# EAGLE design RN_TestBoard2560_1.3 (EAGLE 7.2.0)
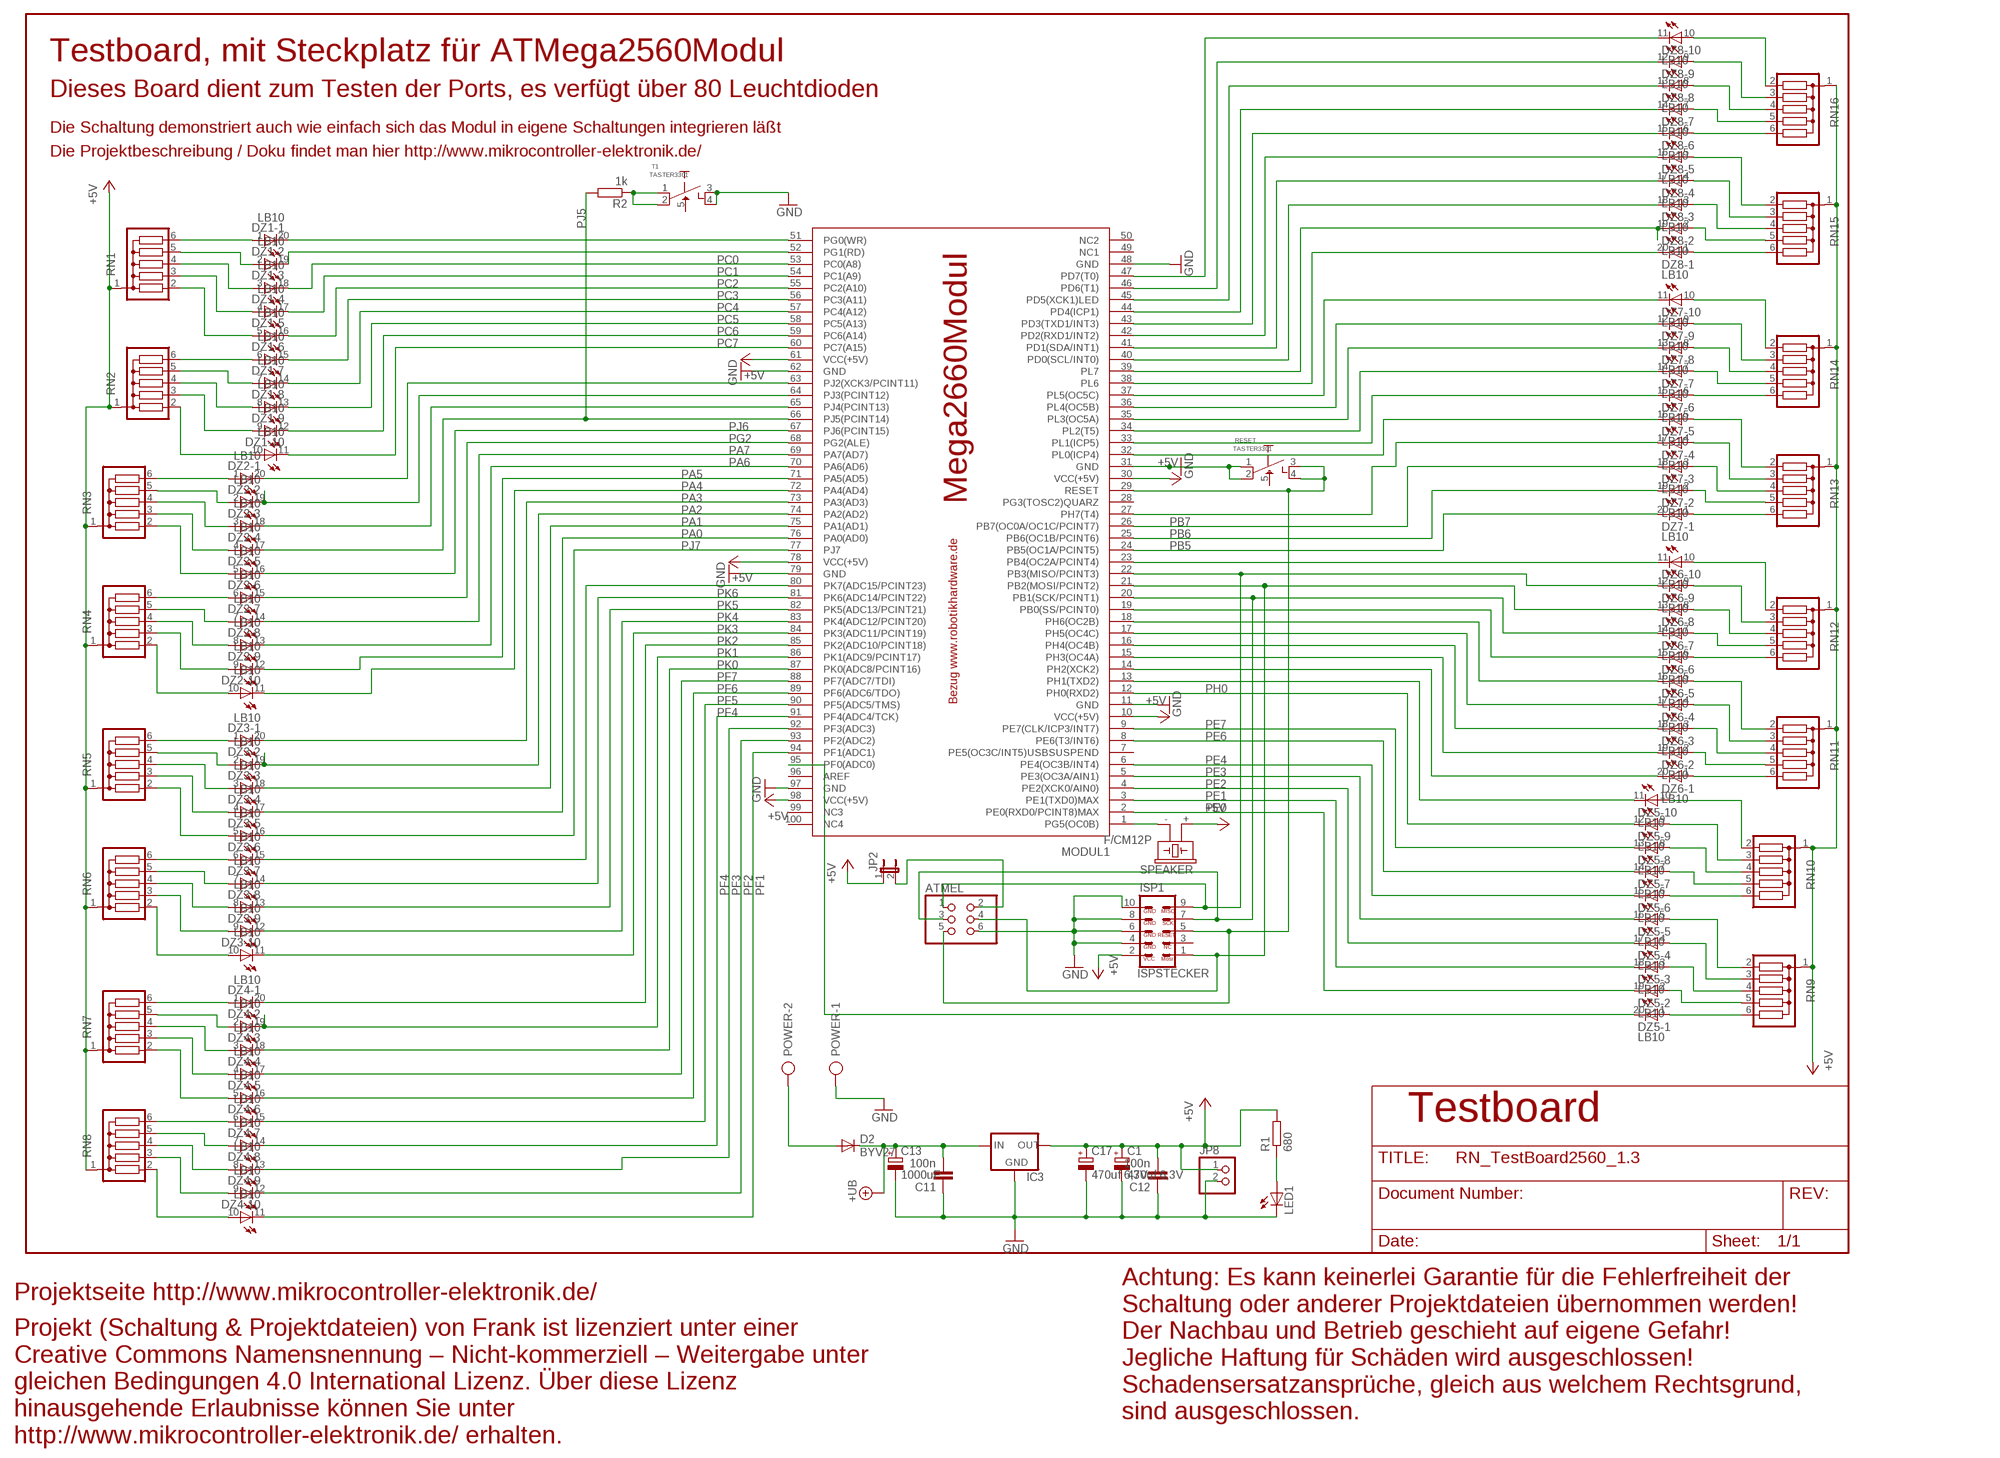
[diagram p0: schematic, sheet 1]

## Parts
ATMEL  PINHD-2X3  [2X03]
C1  470uf 6,3V  CPOL-EUE3.5-8  [E3,5-8]
C11  100n  C-EU050-024X044  [C050-024X044]
C12  100n  C-EU050-024X044  [C050-024X044]
C13  1000uF  CPOL-EUE5-13  [E5-13]
C17  470uf 6,3V  CPOL-EUE3.5-8  [E3,5-8]
D2  BYV27  [SOD57-10]
DZ1  LB10  [LB10]
DZ2  LB10  [LB10]
DZ3  LB10  [LB10]
DZ4  LB10  [LB10]
DZ5  LB10  [LB10]
DZ6  LB10  [LB10]
DZ7  LB10  [LB10]
DZ8  LB10  [LB10]
IC3  78XXS  [78XXS]
ISP1  ISPSTECKER  [ML10]
JP2  JP1E  [JP1]
JP8  PINHD-1X2  [1X02]
LED1  LED3MM  [LED3MM]
MODUL1  MEGA2560MODUL  [MEGA2560MODUL]
POWER  AK500/2  [AK500/2]
R1  680  R-EU_0207/10  [0207/10]
R2  1k  R-EU_0207/10  [0207/10]
RESET  TASTER3301  [TASTER]
RN1  G05R  [SIL6]
RN2  G05R  [SIL6]
RN3  G05R  [SIL6]
RN4  G05R  [SIL6]
RN5  G05R  [SIL6]
RN6  G05R  [SIL6]
RN7  G05R  [SIL6]
RN8  G05R  [SIL6]
RN9  G05R  [SIL6]
RN10  G05R  [SIL6]
RN11  G05R  [SIL6]
RN12  G05R  [SIL6]
RN13  G05R  [SIL6]
RN14  G05R  [SIL6]
RN15  G05R  [SIL6]
RN16  G05R  [SIL6]
SPEAKER  F/CM12P  [F/CM12P]
T1  TASTER3301  [TASTER]

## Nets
+5V [Power3A]: C1.+ C12.2 C17.+ IC3.OUT ISP1.2 JP2.1 JP8.1 MODUL1.10(VCC(+5V)) MODUL1.30(VCC(+5V)) MODUL1.61(VCC(+5V)) MODUL1.78(VCC(+5V)) MODUL1.98(VCC(+5V)) R1.2 RN1.1 RN2.1 RN3.1 RN4.1 RN5.1 RN6.1 RN7.1 RN8.1 RN9.1 RN10.1 RN11.1 RN12.1 RN13.1 RN14.1 RN15.1 RN16.1 SPEAKER.+
+UB [Power2A]: C11.2 C13.+ D2.C IC3.IN
GND [Power2A]: ATMEL.6 C1.- C11.1 C12.1 C13.- C17.- IC3.GND ISP1.4 ISP1.6 ISP1.8 ISP1.10 JP8.2 LED1.K(C) MODUL1.11(GND) MODUL1.31(GND) MODUL1.48(GND) MODUL1.62(GND) MODUL1.79(GND) MODUL1.97(GND) POWER.1 RESET.1 RESET.2 T1.3 T1.4
N$1: ATMEL.2 JP2.2
N$2: ATMEL.5 ISP1.5 MODUL1.29(RESET) RESET.3 RESET.4
N$3: DZ5.20(-1:C) MODUL1.95(PF0(ADC0))
N$4: LED1.A R1.1
N$5: R2.1 T1.1 T1.2
N$9: DZ1.1(-1:A) RN1.6
N$10: DZ1.2(-2:A) RN1.5
N$11: DZ1.3(-3:A) RN1.4
N$12: DZ1.4(-4:A) RN1.3
N$13: DZ1.5(-5:A) RN1.2
N$14: DZ1.6(-6:A) RN2.6
N$15: DZ1.7(-7:A) RN2.5
N$16: DZ1.8(-8:A) RN2.4
N$17: DZ1.9(-9:A) RN2.3
N$18: DZ1.10(-10:A) RN2.2
N$19: DZ1.20(-1:C) MODUL1.51(PG0(WR))
N$20: DZ1.19(-2:C) MODUL1.52(PG1(RD))
N$29: DZ2.3(-3:A) RN3.4
N$30: DZ2.4(-4:A) RN3.3
N$31: DZ2.5(-5:A) RN3.2
N$32: DZ2.7(-7:A) RN4.5
N$33: DZ2.8(-8:A) RN4.4
N$34: DZ2.9(-9:A) RN4.3
N$35: DZ2.10(-10:A) RN4.2
N$36: DZ2.18(-3:C) MODUL1.65(PJ4(PCINT13))
N$37: D2.A POWER.2
N$45: DZ2.1(-1:A) RN3.6
N$46: DZ2.2(-2:A) RN3.5
N$47: DZ2.6(-6:A) RN4.6
N$48: DZ2.20(-1:C) MODUL1.63(PJ2(XCK3/PCINT11))
N$49: DZ2.19(-2:C) MODUL1.64(PJ3(PCINT12))
N$50: DZ8.16(-5:C) MODUL1.42(PD2(RXD1/INT2))
N$52: DZ5.3(-3:A) RN9.4
N$53: DZ5.4(-4:A) RN9.3
N$54: DZ5.5(-5:A) RN9.2
N$55: DZ5.7(-7:A) RN10.5
N$56: DZ5.8(-8:A) RN10.4
N$57: MODUL1.1(PG5(OC0B)) SPEAKER.-
N$58: DZ5.9(-9:A) RN10.3
N$59: DZ3.3(-3:A) RN5.4
N$60: DZ3.4(-4:A) RN5.3
N$61: DZ3.5(-5:A) RN5.2
N$62: DZ3.7(-7:A) RN6.5
N$63: DZ3.8(-8:A) RN6.4
N$64: DZ3.9(-9:A) RN6.3
N$65: DZ3.10(-10:A) RN6.2
N$69: DZ3.15(-6:C) MODUL1.80(PK7(ADC15/PCINT23))
N$74: DZ3.1(-1:A) RN5.6
N$75: DZ3.2(-2:A) RN5.5
N$76: DZ3.6(-6:A) RN6.6
N$79: DZ5.10(-10:A) RN10.2
N$86: DZ5.11(-10:C) MODUL1.13(PH1(TXD2))
N$87: DZ6.20(-1:C) MODUL1.14(PH2(XCK2))
N$88: DZ5.1(-1:A) RN9.6
N$89: DZ4.3(-3:A) RN7.4
N$90: DZ4.4(-4:A) RN7.3
N$91: DZ4.5(-5:A) RN7.2
N$92: DZ4.7(-7:A) RN8.5
N$93: DZ4.8(-8:A) RN8.4
N$94: DZ4.9(-9:A) RN8.3
N$95: DZ4.10(-10:A) RN8.2
N$104: DZ4.1(-1:A) RN7.6
N$105: DZ4.2(-2:A) RN7.5
N$106: DZ4.6(-6:A) RN8.6
N$109: DZ5.2(-2:A) RN9.5
N$110: DZ5.6(-6:A) RN10.6
N$113: DZ6.3(-3:A) RN11.4
N$114: DZ6.4(-4:A) RN11.3
N$115: DZ6.5(-5:A) RN11.2
N$116: DZ6.7(-7:A) RN12.5
N$117: DZ6.8(-8:A) RN12.4
N$118: DZ6.9(-9:A) RN12.3
N$119: DZ6.10(-10:A) RN12.2
N$120: DZ6.17(-4:C) MODUL1.17(PH5(OC4C))
N$121: DZ6.16(-5:C) MODUL1.18(PH6(OC2B))
N$122: DZ6.15(-6:C) MODUL1.19(PB0(SS/PCINT0))
N$123: ATMEL.3 DZ6.14(-7:C) ISP1.7 MODUL1.20(PB1(SCK/PCINT1))
N$124: ATMEL.4 DZ6.13(-8:C) ISP1.1 MODUL1.21(PB2(MOSI/PCINT2))
N$125: ATMEL.1 DZ6.12(-9:C) ISP1.9 MODUL1.22(PB3(MISO/PCINT3))
N$126: DZ6.11(-10:C) MODUL1.23(PB4(OC2A/PCINT4))
N$128: DZ6.1(-1:A) RN11.6
N$129: DZ6.2(-2:A) RN11.5
N$130: DZ6.6(-6:A) RN12.6
N$131: DZ6.18(-3:C) MODUL1.16(PH4(OC4B))
N$132: DZ6.19(-2:C) MODUL1.15(PH3(OC4A))
N$133: DZ7.3(-3:A) RN13.4
N$134: DZ7.4(-4:A) RN13.3
N$135: DZ7.5(-5:A) RN13.2
N$136: DZ7.7(-7:A) RN14.5
N$137: DZ7.8(-8:A) RN14.4
N$138: DZ7.9(-9:A) RN14.3
N$139: DZ7.10(-10:A) RN14.2
N$140: DZ7.17(-4:C) MODUL1.27(PH7(T4))
N$142: DZ7.16(-5:C) MODUL1.32(PL0(ICP4))
N$143: DZ7.15(-6:C) MODUL1.33(PL1(ICP5))
N$144: DZ7.14(-7:C) MODUL1.34(PL2(T5))
N$145: DZ7.13(-8:C) MODUL1.35(PL3(OC5A))
N$146: DZ7.12(-9:C) MODUL1.36(PL4(OC5B))
N$147: DZ7.11(-10:C) MODUL1.37(PL5(OC5C))
N$148: DZ7.1(-1:A) RN13.6
N$149: DZ7.2(-2:A) RN13.5
N$150: DZ7.6(-6:A) RN14.6
N$153: DZ8.3(-3:A) RN15.4
N$154: DZ8.4(-4:A) RN15.3
N$155: DZ8.5(-5:A) RN15.2
N$156: DZ8.7(-7:A) RN16.5
N$157: DZ8.8(-8:A) RN16.4
N$158: DZ8.9(-9:A) RN16.3
N$159: DZ8.10(-10:A) RN16.2
N$160: DZ8.18(-3:C) MODUL1.40(PD0(SCL/INT0))
N$161: DZ8.17(-4:C) MODUL1.41(PD1(SDA/INT1))
N$163: DZ8.15(-6:C) MODUL1.43(PD3(TXD1/INT3))
N$164: DZ8.14(-7:C) MODUL1.44(PD4(ICP1))
N$165: DZ8.13(-8:C) MODUL1.45(PD5(XCK1)LED)
N$166: DZ8.12(-9:C) MODUL1.46(PD6(T1))
N$167: DZ8.11(-10:C) MODUL1.47(PD7(T0))
N$168: DZ8.1(-1:A) RN15.6
N$169: DZ8.2(-2:A) RN15.5
N$170: DZ8.6(-6:A) RN16.6
N$171: DZ8.19(-2:C) MODUL1.39(PL7)
N$172: DZ8.20(-1:C) MODUL1.38(PL6)
PA0: DZ3.17(-4:C) MODUL1.76(PA0(AD0))
PA1: DZ3.18(-3:C) MODUL1.75(PA1(AD1))
PA2: DZ3.19(-2:C) MODUL1.74(PA2(AD2))
PA3: DZ3.20(-1:C) MODUL1.73(PA3(AD3))
PA4: DZ2.11(-10:C) MODUL1.72(PA4(AD4))
PA5: DZ2.12(-9:C) MODUL1.71(PA5(AD5))
PA6: DZ2.13(-8:C) MODUL1.70(PA6(AD6))
PA7: DZ2.14(-7:C) MODUL1.69(PA7(AD7))
PB5: DZ7.20(-1:C) MODUL1.24(PB5(OC1A/PCINT5))
PB6: DZ7.19(-2:C) MODUL1.25(PB6(OC1B/PCINT6))
PB7: DZ7.18(-3:C) MODUL1.26(PB7(OC0A/OC1C/PCINT7))
PC0: DZ1.18(-3:C) MODUL1.53(PC0(A8))
PC1: DZ1.17(-4:C) MODUL1.54(PC1(A9))
PC2: DZ1.16(-5:C) MODUL1.55(PC2(A10))
PC3: DZ1.15(-6:C) MODUL1.56(PC3(A11))
PC4: DZ1.14(-7:C) MODUL1.57(PC4(A12))
PC5: DZ1.13(-8:C) MODUL1.58(PC5(A13))
PC6: DZ1.12(-9:C) MODUL1.59(PC6(A14))
PC7: DZ1.11(-10:C) MODUL1.60(PC7(A15))
PE0: DZ5.19(-2:C) MODUL1.2(PE0(RXD0/PCINT8)MAX)
PE1: DZ5.18(-3:C) MODUL1.3(PE1(TXD0)MAX)
PE2: DZ5.17(-4:C) MODUL1.4(PE2(XCK0/AIN0))
PE3: DZ5.16(-5:C) MODUL1.5(PE3(OC3A/AIN1))
PE4: DZ5.15(-6:C) MODUL1.6(PE4(OC3B/INT4))
PE6: DZ5.14(-7:C) MODUL1.8(PE6(T3/INT6))
PE7: DZ5.13(-8:C) MODUL1.9(PE7(CLK/ICP3/INT7))
PF1: DZ4.11(-10:C) MODUL1.94(PF1(ADC1))
PF2: DZ4.12(-9:C) MODUL1.93(PF2(ADC2))
PF3: DZ4.13(-8:C) MODUL1.92(PF3(ADC3))
PF4: DZ4.14(-7:C) MODUL1.91(PF4(ADC4/TCK))
PF5: DZ4.15(-6:C) MODUL1.90(PF5(ADC5/TMS))
PF6: DZ4.16(-5:C) MODUL1.89(PF6(ADC6/TDO))
PF7: DZ4.17(-4:C) MODUL1.88(PF7(ADC7/TDI))
PG2: DZ2.15(-6:C) MODUL1.68(PG2(ALE))
PH0: DZ5.12(-9:C) MODUL1.12(PH0(RXD2))
PJ5: DZ2.17(-4:C) MODUL1.66(PJ5(PCINT14)) R2.2
PJ6: DZ2.16(-5:C) MODUL1.67(PJ6(PCINT15))
PJ7: DZ3.16(-5:C) MODUL1.77(PJ7)
PK0: DZ4.18(-3:C) MODUL1.87(PK0(ADC8/PCINT16))
PK1: DZ4.19(-2:C) MODUL1.86(PK1(ADC9/PCINT17))
PK2: DZ4.20(-1:C) MODUL1.85(PK2(ADC10/PCINT18))
PK3: DZ3.11(-10:C) MODUL1.84(PK3(ADC11/PCINT19))
PK4: DZ3.12(-9:C) MODUL1.83(PK4(ADC12/PCINT20))
PK5: DZ3.13(-8:C) MODUL1.82(PK5(ADC13/PCINT21))
PK6: DZ3.14(-7:C) MODUL1.81(PK6(ADC14/PCINT22))
Unconnected: ISP1.3 MODUL1.7(PE5(OC3C/INT5)USBSUSPEND) MODUL1.28(PG3(TOSC2)QUARZ) MODUL1.49(NC1) MODUL1.50(NC2) MODUL1.96(AREF) MODUL1.99(NC3) MODUL1.100(NC4) RESET.5 T1.5

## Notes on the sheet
- Testboard, mit Steckplatz für ATMega2560Modul
- Dieses Board dient zum Testen der Ports, es verfügt über 80 Leuchtdioden
- Die Schaltung demonstriert auch wie einfach sich das Modul in eigene Schaltungen integrieren läßt
- Die Projektbeschreibung / Doku findet man hier http://www.mikrocontroller-elektronik.de/
- Testboard
- Projektseite http://www.mikrocontroller-elektronik.de/
- Achtung: Es kann keinerlei Garantie für die Fehlerfreiheit der
  Schaltung oder anderer Projektdateien übernommen werden!
  Der Nachbau und Betrieb geschieht auf eigene Gefahr! 
  Jegliche Haftung für Schäden wird ausgeschlossen!
  Schadensersatzansprüche, gleich aus welchem Rechtsgrund,
  sind ausgeschlossen.
- Projekt (Schaltung & Projektdateien) von Frank ist lizenziert unter einer
  Creative Commons Namensnennung – Nicht-kommerziell – Weitergabe unter
  gleichen Bedingungen 4.0 International Lizenz. Über diese Lizenz
  hinausgehende Erlaubnisse können Sie unter
  http://www.mikrocontroller-elektronik.de/ erhalten.

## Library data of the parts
ATMEL = pinhead:PINHD-2X3: PIN HEADER
C1 C13 C17 = rcl:CPOL-EU: POLARIZED CAPACITOR, European symbol
C11 C12 = rcl:C-EU: CAPACITOR, European symbol
D2 = diode:BYV27: DIODE
DZ1-DZ8 = led:LB10: LED BLOCK 10-LED bar graph, DIL, Siemens
IC3 = v-reg:78XXS: VOLTAGE REGULATOR
ISP1 = RoboterNetz:ISPSTECKER
JP2 = jumper:JP1E: JUMPER
JP8 = pinhead:PINHD-1X2: PIN HEADER
LED1 = led:LED: LED
MODUL1 = RoboterNetz:MEGA2560MODUL: Sehr kleines Modul mit leistungsstarkem AVR AtMega2560 Controller , RS232 als auch USB - Schnittstelle. Bestückt auch mit Standard ISP Wannenstiftleiste Stecker zum programmieren. Durch modernste SMD Bauteile konnte das Modul so klein gehalten werden. Der Pinabstand der beiden Stiftleisten ist so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
POWER = con-ptr500:AK500/2: CONNECTOR
R1 R2 = rcl:R-EU_: RESISTOR, European symbol
RESET T1 = RoboterNetz:TASTER3301: Taster 3301 Bezugsquelle z.B. Reichelt
RN1-RN16 = resistor-sil:G05R: SIL RESISTOR
SPEAKER = buzzer:F/CM12P: BUZZER

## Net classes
1 power: width 0.457 mm
2 Power2A: width 0.762 mm
3 Power3A: width 1.016 mm

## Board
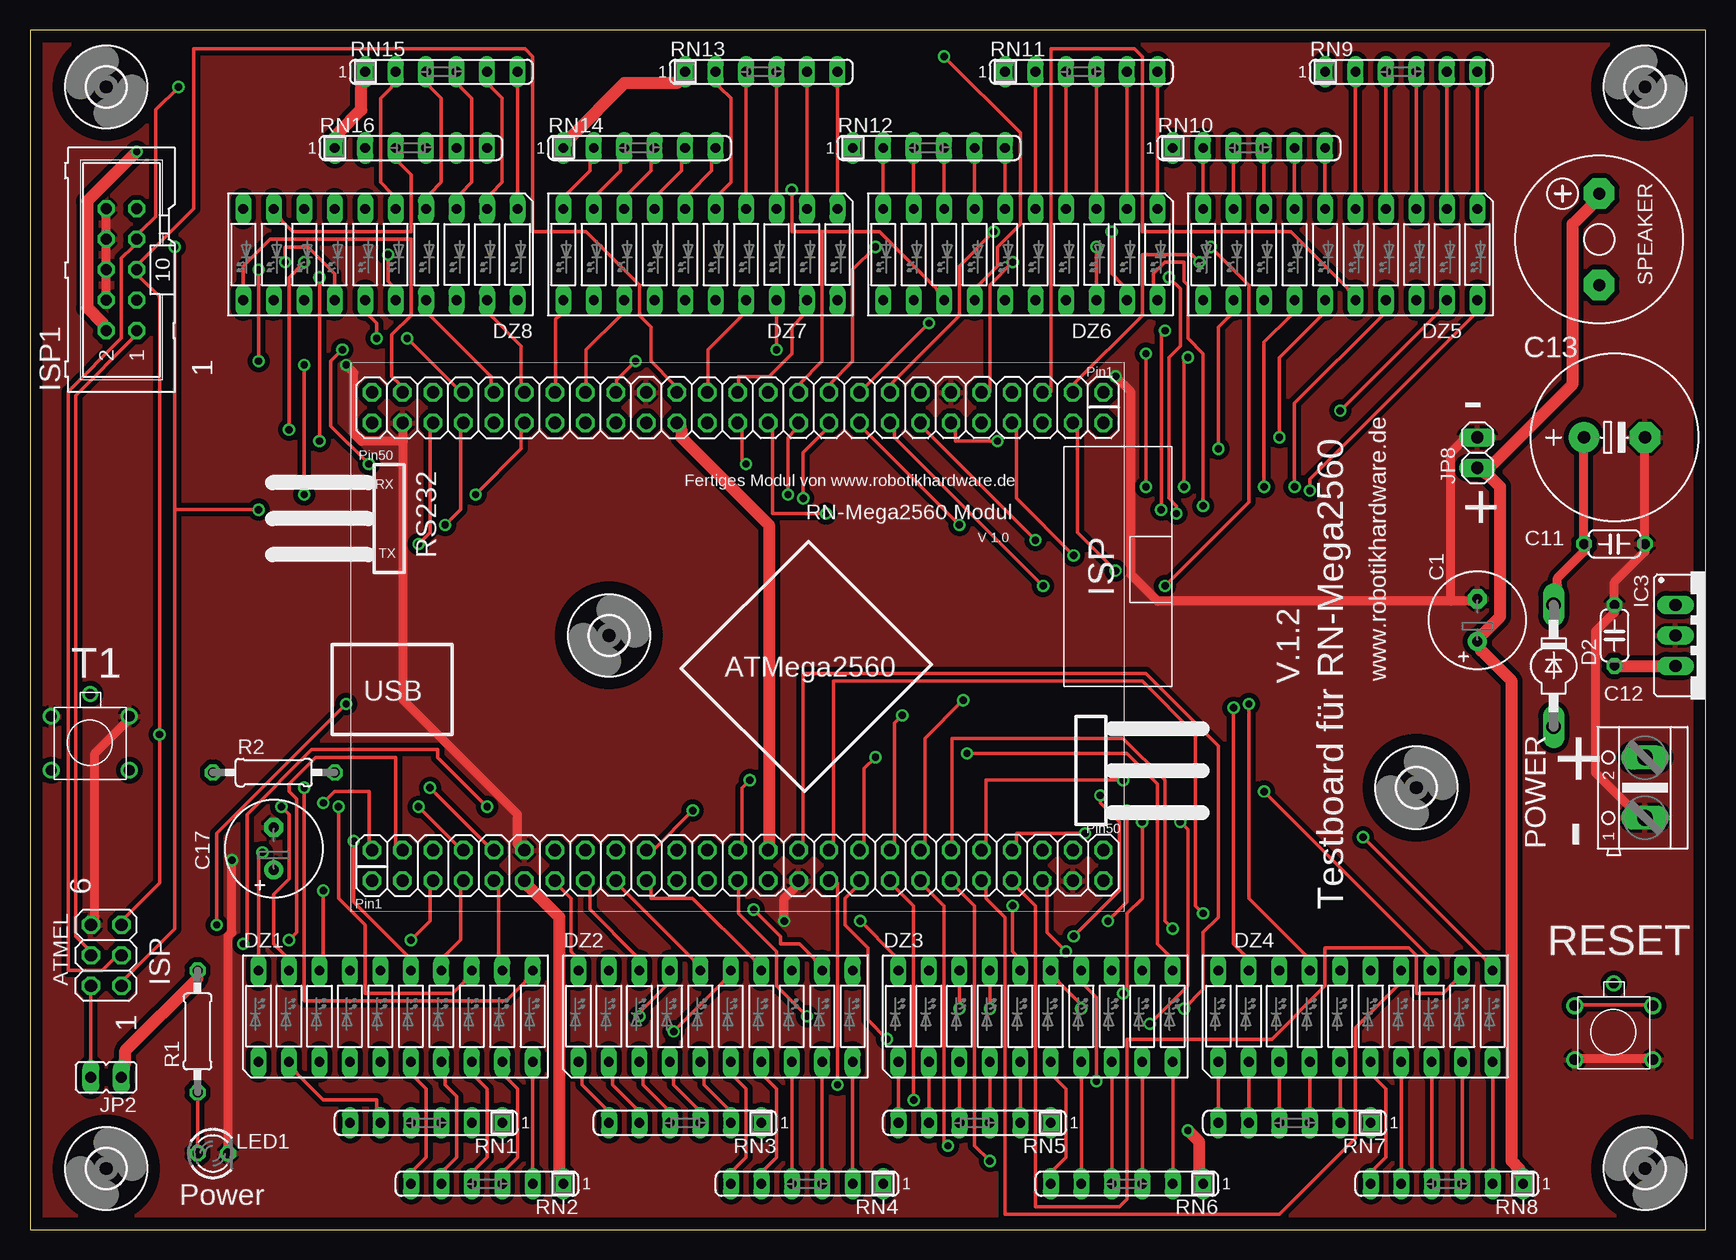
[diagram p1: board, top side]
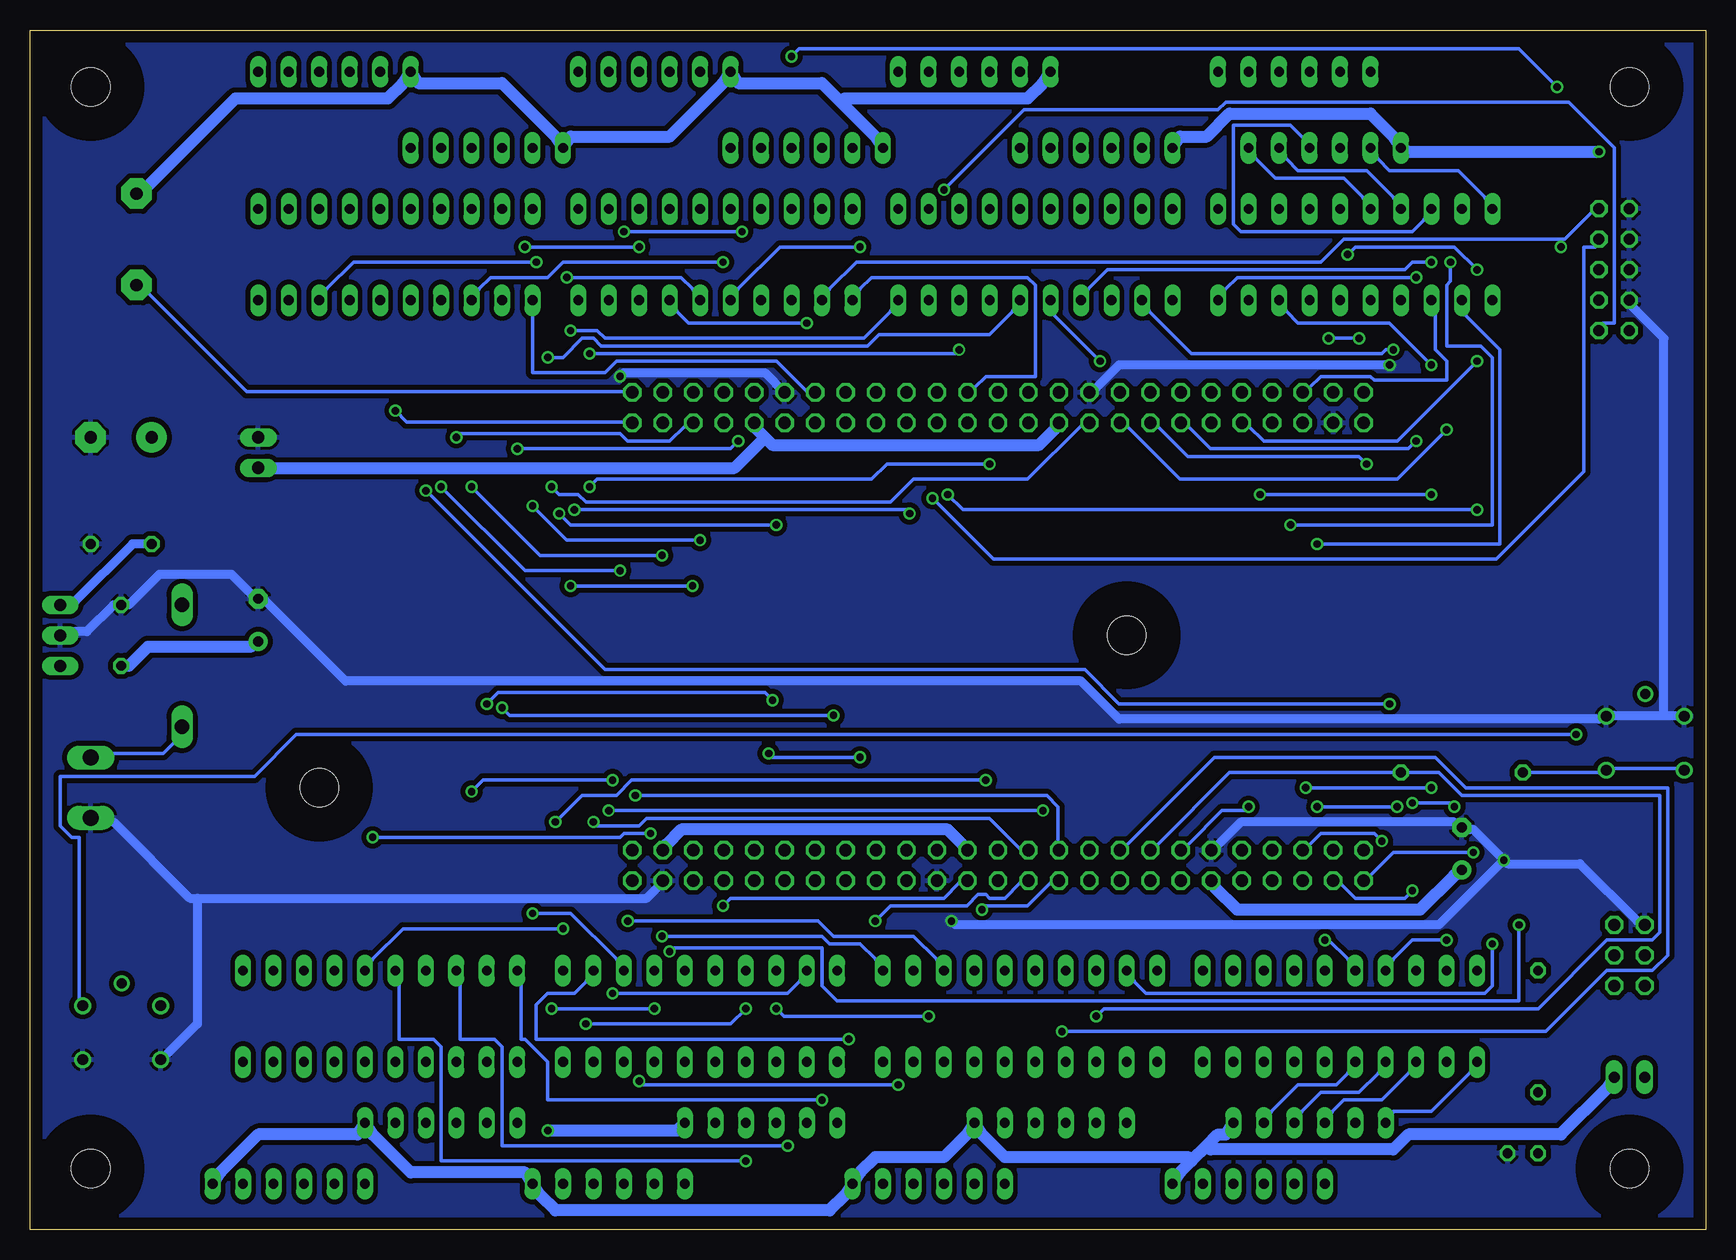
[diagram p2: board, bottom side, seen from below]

Size 139.68 x 100 mm. Coordinates in mm from the lower left corner, seen from the top.
Outline: 0,0 139.68,0 139.68,100 0,100 0,0
Copper layers (1*16): Top 0.035mm / dielectric 1.5mm / Bottom 0.035mm
Design rules "default": minimum track width 12mil, minimum drill 24mil, track to track 8mil, track to pad 12mil, pad to pad 8mil, via to via 8mil, smd to smd 8mil, copper to edge 40mil, drill to drill 8mil, minimum pad ring 10mil, minimum via ring 8mil, stop-mask expansion 4mil, vias tented up to drill 0mil, thermal gap 10mil

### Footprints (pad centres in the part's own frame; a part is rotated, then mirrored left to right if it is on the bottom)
2X03 = drill 1.016 octagon: 1 -2.54,-1.27; 2 -2.54,1.27; 3 0,-1.27; 4 0,1.27; 5 2.54,-1.27; 6 2.54,1.27
E3,5-8 = drill 0.813 pad 1.6: + -1.778,0 | drill 0.813 pad 1.6 octagon: - 1.778,0
C050-024X044 = drill 0.813 octagon: 1 -2.54,0; 2 2.54,0
E5-13 = drill 1.016 pad 2.54: + -2.54,0 | drill 1.016 pad 2.54 octagon: - 2.54,0
SOD57-10 = drill 1.194 long: A 5.08,0; C -5.08,0
LB10 = drill 0.813 long: 1 -11.43,-3.81; 2 -8.89,-3.81; 3 -6.35,-3.81; 4 -3.81,-3.81; 5 -1.27,-3.81; 6 1.27,-3.81; 7 3.81,-3.81; 8 6.35,-3.81; 9 8.89,-3.81; 10 11.43,-3.81; 11 11.43,3.81; 12 8.89,3.81; 13 6.35,3.81; 14 3.81,3.81; 15 1.27,3.81; 16 -1.27,3.81; 17 -3.81,3.81; 18 -6.35,3.81; 19 -8.89,3.81; 20 -11.43,3.81
78XXS = drill 1.016 long: GND 0,-2.54; IN -2.54,-2.54; OUT 2.54,-2.54
ML10 = drill 0.914 octagon: 1 -5.08,-1.27; 2 -5.08,1.27; 3 -2.54,-1.27; 4 -2.54,1.27; 5 0,-1.27; 6 0,1.27; 7 2.54,-1.27; 8 2.54,1.27; 9 5.08,-1.27; 10 5.08,1.27
JP1 = drill 0.914 long: 1 0,-1.27; 2 0,1.27
1X02 = drill 1.016 long: 1 -1.27,0; 2 1.27,0
LED3MM = drill 0.813 octagon: A -1.27,0; K 1.27,0
MEGA2560MODUL = drill 1.016 octagon: 1 -29.782,-21.526; 2 -29.782,-18.986; 3 -27.241,-21.526; 4 -27.241,-18.986; 5 -24.701,-21.526; 6 -24.701,-18.986; 7 -22.162,-21.526; 8 -22.162,-18.986; 9 -19.622,-21.526; 10 -19.622,-18.986; 11 -17.081,-21.526; 12 -17.081,-18.986; 13 -14.541,-21.526; 14 -14.541,-18.986; 15 -12.002,-21.526; 16 -12.002,-18.986; 17 -9.461,-21.526; 18 -9.461,-18.986; 19 -6.921,-21.526; 20 -6.921,-18.986; 21 -4.381,-21.526; 22 -4.381,-18.986; 23 -1.841,-21.526; 24 -1.841,-18.986; 25 0.699,-21.526; 26 0.699,-18.986; 27 3.239,-21.526; 28 3.239,-18.986; 29 5.779,-21.526; 30 5.779,-18.986; 31 8.319,-21.526; 32 8.319,-18.986; 33 10.858,-21.526; 34 10.858,-18.986; 35 13.399,-21.526; 36 13.399,-18.986; 37 15.938,-21.526; 38 15.938,-18.986; 39 18.479,-21.526; 40 18.479,-18.986; 41 21.018,-21.526; 42 21.018,-18.986; 43 23.558,-21.526; 44 23.558,-18.986; 45 26.099,-21.526; 46 26.099,-18.986; 47 28.639,-21.526; 48 28.639,-18.986; 49 31.178,-21.526; 50 31.178,-18.986; 51 31.178,19.177; 52 31.178,16.637; 53 28.639,19.177; 54 28.639,16.637; 55 26.099,19.177; 56 26.099,16.637; 57 23.558,19.177; 58 23.558,16.637; 59 21.018,19.177; 60 21.018,16.637; 61 18.479,19.177; 62 18.479,16.637; 63 15.938,19.177; 64 15.938,16.637; 65 13.399,19.177; 66 13.399,16.637; 67 10.858,19.177; 68 10.858,16.637; 69 8.319,19.177; 70 8.319,16.637; 71 5.779,19.177; 72 5.779,16.637; 73 3.239,19.177; 74 3.239,16.637; 75 0.699,19.177; 76 0.699,16.637; 77 -1.841,19.177; 78 -1.841,16.637; 79 -4.381,19.177; 80 -4.381,16.637; 81 -6.921,19.177; 82 -6.921,16.637; 83 -9.461,19.177; 84 -9.461,16.637; 85 -12.002,19.177; 86 -12.002,16.637; 87 -14.541,19.177; 88 -14.541,16.637; 89 -17.081,19.177; 90 -17.081,16.637; 91 -19.622,19.177; 92 -19.622,16.637; 93 -22.162,19.177; 94 -22.162,16.637; 95 -24.701,19.177; 96 -24.701,16.637; 97 -27.241,19.177; 98 -27.241,16.637; 99 -29.782,19.177; 100 -29.782,16.637
AK500/2 = drill 1.321 long: 1 -2.515,0; 2 2.515,0
0207/10 = drill 0.813 octagon: 1 -5.08,0; 2 5.08,0
TASTER = drill 0.9: 1 -2.35,-3.2; 2 -2.35,3.3; 3 2.15,-3.2; 4 2.15,3.3 | drill 0.813: 5 4.005,0.055
SIL6 = drill 0.813 long: 1 -6.35,0; 2 -3.81,0; 3 -1.27,0; 4 1.27,0; 5 3.81,0; 6 6.35,0
F/CM12P = drill 1.016 pad 2.54 octagon: + 3.81,0; - -3.81,0
3,2 = hole 3.2: 0,0

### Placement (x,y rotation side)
ATMEL  6.35,22.86 90 top
C1  120.65,50.8 90 top
C11  132.08,57.15 180 top
C12  132.08,49.53 270 top
C13  132.08,66.04 0 top
C17  20.32,31.75 90 top
D2  127,46.99 270 top
DZ1  30.48,17.78 0 top
DZ2  57.15,17.78 0 top
DZ3  83.82,17.78 0 top
DZ4  110.49,17.78 0 top
DZ5  109.22,81.28 180 top
DZ6  82.55,81.28 180 top
DZ7  55.88,81.28 180 top
DZ8  29.21,81.28 180 top
IC3  139.7,49.53 270 top
ISP1  7.62,80.01 90 top
JP2  6.35,12.7 90 top
JP8  120.65,64.77 90 top
LED1  15.24,6.35 0 top
MODUL1  59.69,48.26 180 top
POWER  134.62,36.83 90 top
R1  13.97,16.51 90 top
R2  20.32,38.1 0 top
RESET  132.08,16.51 90 top
RN1  33.02,8.89 180 top
RN2  38.1,3.81 180 top
RN3  54.61,8.89 180 top
RN4  64.77,3.81 180 top
RN5  78.74,8.89 180 top
RN6  91.44,3.81 180 top
RN7  105.41,8.89 180 top
RN8  118.11,3.81 180 top
RN9  114.3,96.52 0 top
RN10  101.6,90.17 0 top
RN11  87.63,96.52 0 top
RN12  74.93,90.17 0 top
RN13  60.96,96.52 0 top
RN14  50.8,90.17 0 top
RN15  34.29,96.52 0 top
RN16  31.75,90.17 0 top
SPEAKER  130.81,82.55 90 top
T1  5.08,40.64 90 top
U$1  [3,2]  6.35,5.08 0 top
U$2  [3,2]  6.35,95.25 90 top
U$3  [3,2]  134.62,5.08 90 top
U$4  [3,2]  115.57,36.83 0 top
U$5  [3,2]  134.62,95.25 90 top
U$6  [3,2]  48.26,49.53 0 top

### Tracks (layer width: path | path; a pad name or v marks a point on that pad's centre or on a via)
+5V  (via drill 0.61)
  Top 1.016: v96.52,8.26 97.47,7.3 97.47,5.08 RN6.1 | R1.2 13.97,20.95 7.94,14.92 7.94,13.97 JP2.1 | MODUL1.61 41.59,28.57 44.13,26.04 44.13,5.08 RN2.1 | MODUL1.78 61.59,32.07 61.59,58.74 54.29,66.04 54.29,66.67 MODUL1.30 | RN16.1 25.72,91.44 27.62,93.34 27.62,95.25 RN15.1 | v8.89,89.85 4.76,85.72 4.76,76.83 6.03,75.56 ISP1.2 | RN14.1 45.09,91.12 49.53,95.57 53.98,95.57 RN13.1 | C12.2 IC3.OUT | SPEAKER.+ 130.18,85.41 128.59,83.82 128.59,70.48 121.92,63.82 JP8.1 121.6,62.87 122.56,61.91 122.56,51.12 120.97,49.53 C1.+ 120.97,48.26 123.51,45.72 123.51,5.71 124.14,5.08 RN8.1
  Bottom 1.016: v96.52,8.26 85.72,8.26 RN5.1 | RN8.1 123.83,4.76 120.65,7.94 112.39,7.94 RN7.1 111.12,7.94 107.95,4.76 98.42,4.76 RN6.1 97.16,2.86 95.89,1.59 73.03,1.59 71.75,2.86 RN4.1 70.48,4.76 69.22,6.03 63.5,6.03 61.59,7.94 RN3.1 60.33,7.94 58.42,6.03 43.18,6.03 42.86,5.71 | 41.59,6.99 40.64,7.94 40.01,7.94 RN1.1 | 41.59,6.99 42.86,5.71 | 42.86,5.71 43.81,4.76 RN2.1 | C17.+ 20.95,29.53 23.81,26.67 39.05,26.67 40.96,28.57 MODUL1.61 | JP2.1 8.26,11.75 12.06,7.94 24.77,7.94 26.04,6.67 41.27,6.67 41.59,6.99 | MODUL1.78 61.91,32.07 63.18,33.34 85.41,33.34 86.68,32.07 MODUL1.98 | 78.42,66.04 79.06,66.67 MODUL1.10 | 78.42,66.04 77.79,65.41 55.56,65.41 54.29,66.67 MODUL1.30 | v8.89,89.85 24.77,89.85 RN16.1 26.04,91.12 27.94,93.03 39.69,93.03 41.59,91.12 43.81,91.12 RN14.1 | 72.07,93.98 73.66,95.57 80.64,95.57 RN11.1 81.92,95.57 86.36,91.12 94.61,91.12 RN10.1 95.89,91.12 100.33,95.57 107.31,95.57 RN9.1 108.58,95.57 109.86,94.3 122.56,94.3 129.86,87 SPEAKER.+ | 72.07,93.98 69.22,91.12 RN12.1 | RN13.1 55.24,95.57 56.52,94.3 71.75,94.3 72.07,93.98 | C12.2 131.44,46.99 129.86,48.58 121.28,48.58 C1.+ | 78.42,66.04 80.96,63.5 JP8.1
+UB
  Top 0.762: D2.C 127.32,53.66 127.32,54.29 129.54,56.52 C11.2 C13.+
  Bottom 0.762: IC3.IN 135.89,52.39 131.13,57.15 C11.2
GND  (via drill 0.61)
  Top 0.762: RESET.2 129.22,14.29 134.62,14.29 RESET.1 | C13.- C11.1 134.62,56.52 132.08,53.98 C12.1 132.08,51.44 130.49,49.85 130.49,38.1 133.35,35.24 POWER.1 | v90.49,71.12 91.76,69.85 91.76,54.61 93.98,52.39 118.43,52.39 | 118.43,52.39 120.02,52.39 C1.- | JP8.2 119.38,65.72 118.43,64.77 118.43,52.39 | ISP1.4 ISP1.6 ISP1.8 ISP1.10 | v16.83,30.8 16.83,24.77 16.51,24.45 LED1.K | 31.11,65.72 31.11,44.13 40.64,34.61 40.64,32.07 MODUL1.62 | 31.11,65.72 31.11,66.67 MODUL1.48 | v62.87,25.72 62.87,27.62 63.82,28.57 MODUL1.79 | v26.35,72.07 26.99,71.44 26.99,66.36 27.62,65.72 31.11,65.72 | T1.3 7.94,42.23 5.4,39.69 5.4,26.04 ATMEL.6
  Bottom 0.762: 125.73,27.62 126.36,27.62 132.72,33.97 POWER.1 | 125.73,27.62 88.27,27.62 87.31,28.57 MODUL1.97 | RESET.2 128.27,14.61 125.73,17.14 125.73,27.62 | IC3.GND 135.89,49.85 134.94,49.85 132.72,52.07 C12.1 131.44,52.07 128.91,54.61 122.87,54.61 121.28,53.02 C1.- 120.02,52.39 113.35,45.72 52.07,45.72 48.9,42.55 8.89,42.55 T1.3 7.62,42.86 3.49,42.86 | v90.49,71.12 90.17,71.44 78.42,71.44 MODUL1.11 | 3.49,42.86 2.22,42.86 T1.4 | v16.83,30.8 19.37,33.34 19.68,33.34 C17.- 20.95,33.97 38.73,33.97 40.64,32.07 MODUL1.62 | ATMEL.6 5.71,25.72 10.48,30.48 16.51,30.48 v16.83,30.8 | v62.87,25.72 62.55,25.4 22.23,25.4 v16.83,30.8 | v26.35,72.07 48.9,72.07 50.8,70.17 MODUL1.31 | ISP1.4 6.03,76.83 3.49,74.3 3.49,42.86
  pour Top (isolate 0.406): 0,0 0,99.06 139.7,99.06 139.7,0
  pour Bottom (isolate 0.406): 0,0 0,99.06 139.7,99.06 139.7,0
N$1
  Top 0.305: JP2.2 ATMEL.2
N$2  (via drill 0.61)
  Top 0.305: RESET.4 129.22,18.73 134.62,18.73 RESET.3 | ATMEL.5 7.94,26.04 10.79,28.89 v10.79,41.27 10.79,77.79 9.21,79.38 ISP1.5 9.21,80.64 13.65,85.09 13.65,98.42 41.27,98.42 41.91,97.79 41.91,83.19 46.35,83.19 50.8,78.74 50.8,76.2 51.75,75.25 51.75,72.39 53.66,70.48 MODUL1.29
  Bottom 0.305: v10.79,41.27 117.47,41.27 120.97,37.78 137.16,37.78 137.16,33.66 136.21,32.7 135.57,32.7 135.57,19.05 RESET.3
N$3  (via drill 0.61)
  Top 0.305: v106.68,61.59 106.68,62.55 120.33,76.2 DZ5.20 | v26.35,43.81 15.56,33.02 v15.56,25.4 | v86.36,23.18 84.77,24.77 84.77,28.57 MODUL1.95
  Bottom 0.305: v106.68,61.59 91.76,46.67 51.75,46.67 48.9,43.81 v26.35,43.81 | v15.56,25.4 15.56,19.05 72.39,19.05 73.66,20.32 73.66,23.5 86.04,23.5 v86.36,23.18
N$4
  Top 0.305: LED1.A R1.1
N$5
  Bottom 0.305: R2.1 8.89,38.1 T1.1 7.62,38.42 2.22,38.42 T1.2
N$9
  Bottom 0.305: DZ1.1 19.68,13.02 22.86,9.84 26.04,9.84 RN1.6
N$10
  Top 0.305: DZ1.2 22.23,13.02 24.45,10.79 28.89,10.79 28.89,10.16 RN1.5
N$11
  Bottom 0.305: DZ1.3 24.77,13.02 26.99,10.79 30.16,10.79 31.11,9.84 RN1.4
N$12
  Bottom 0.305: DZ1.4 27.3,13.02 28.89,11.43 32.07,11.43 33.66,9.84 RN1.3
N$13
  Bottom 0.305: DZ1.5 29.84,13.02 30.8,12.06 33.97,12.06 36.2,9.84 RN1.2
N$14
  Top 0.305: RN2.6 32.07,5.08 33.02,6.03 33.02,11.75 32.07,12.7 DZ1.6
N$15
  Top 0.305: RN2.5 34.61,5.08 35.56,6.03 35.56,11.11 34.61,12.06 34.61,12.7 DZ1.7
N$16
  Top 0.305: RN2.4 37.15,5.08 38.1,6.03 38.1,11.75 37.15,12.7 DZ1.8
N$17
  Top 0.305: RN2.3 39.69,5.08 40.64,6.03 40.64,11.75 39.69,12.7 DZ1.9
N$18
  Top 0.305: RN2.2 DZ1.10
N$19  (via drill 0.61)
  Top 0.305: v19.37,31.43 19.05,31.11 DZ1.20
  Bottom 0.305: v19.37,31.43 26.04,31.43 27.94,29.53 MODUL1.51
N$20  (via drill 0.61)
  Top 0.305: v20.95,35.24 21.59,34.61 21.59,29.21 20.32,27.94 20.32,23.81 21.27,22.86 DZ1.19 | v24.45,35.56 25.4,36.51 28.26,36.51 28.26,32.07 MODUL1.52
  Bottom 0.305: v20.95,35.24 21.27,35.56 v24.45,35.56
N$29
  Top 0.305: RN3.4 53.02,10.16 51.12,12.06 51.12,12.7 DZ2.3
N$30
  Top 0.305: RN3.3 55.56,10.16 53.66,12.06 53.66,12.7 DZ2.4
N$31
  Top 0.305: RN3.2 58.1,10.16 56.2,12.06 56.2,12.7 DZ2.5
N$32
  Top 0.305: RN4.5 61.28,5.08 62.23,6.03 62.23,11.75 61.28,12.7 DZ2.7
N$33
  Top 0.305: RN4.4 DZ2.8
N$34
  Top 0.305: RN4.3 DZ2.9
N$35
  Top 0.305: RN4.2 DZ2.10
N$36
  Top 0.305: DZ2.18 50.48,22.86 46.67,26.67 46.67,28.57 MODUL1.65
N$37
  Bottom 0.305: D2.A 127.64,40.64 128.59,39.69 132.72,39.69 POWER.2
N$45
  Top 0.305: RN3.6 47.94,10.16 46.04,12.06 46.04,12.7 DZ2.1
N$46
  Top 0.305: RN3.5 50.48,10.16 48.58,12.06 48.58,12.7 DZ2.2
N$47
  Top 0.305: RN4.6 58.74,5.08 59.69,6.03 59.69,11.75 58.74,12.7 DZ2.6
N$48
  Top 0.305: DZ2.20 45.4,22.86 45.09,23.18 45.09,27.62 44.13,28.57 MODUL1.63
N$49  (via drill 0.61)
  Top 0.305: v17.78,23.81 18.1,24.13 18.1,34.61 23.5,40.01 33.97,40.01 33.97,39.37 v38.1,35.24
  Bottom 0.305: v17.78,23.81 17.78,20.32 18.41,19.68 46.67,19.68 47.62,20.64 DZ2.19 | v38.1,35.24 38.42,34.92 40.32,34.92 43.18,32.07 MODUL1.64
N$50  (via drill 0.61)
  Top 0.305: v29.84,81.28 29.84,79.06 30.16,78.74 DZ8.16 | v19.05,72.39 v19.05,80.01
  Bottom 0.305: v29.84,81.28 29.21,81.92 20.95,81.92 v19.05,80.01 | v19.05,72.39 25.72,65.72 36.83,65.72 38.1,66.99 MODUL1.42
N$52
  Top 0.305: DZ5.3 RN9.4
N$53
  Top 0.305: DZ5.4 RN9.3
N$54
  Top 0.305: DZ5.5 RN9.2
N$55
  Top 0.305: DZ5.7 RN10.5
N$56
  Top 0.305: DZ5.8 RN10.4
N$57
  Bottom 0.305: MODUL1.1 90.17,69.85 121.6,69.85 129.86,78.11 SPEAKER.-
N$58
  Top 0.305: DZ5.9 RN10.3
N$59
  Top 0.305: RN5.4 DZ3.3
N$60
  Top 0.305: RN5.3 DZ3.4
N$61
  Top 0.305: RN5.2 DZ3.5
N$62
  Top 0.305: RN6.5 DZ3.7
N$63
  Top 0.305: RN6.4 DZ3.8
N$64
  Top 0.305: RN6.3 DZ3.9
N$65
  Top 0.305: RN6.2 DZ3.10
N$69  (via drill 0.61)
  Top 0.305: v87.63,18.41 87.63,18.73 85.72,20.64 DZ3.15 | v96.2,18.41 97.79,20 97.79,24.77 99.06,26.04 99.06,40.32 93.03,46.35 64.45,46.35 64.45,32.07 MODUL1.80
  Bottom 0.305: v96.2,18.41 v87.63,18.41
N$74
  Top 0.305: RN5.6 DZ3.1
N$75
  Top 0.305: RN5.5 DZ3.2
N$76
  Top 0.305: RN6.6 85.41,5.08 86.36,6.03 86.36,11.75 85.41,12.7 DZ3.6
N$79
  Top 0.305: DZ5.10 RN10.2
N$86
  Bottom 0.305: DZ5.11 97.79,71.44 91.76,71.44 90.81,72.39 77.47,72.39 74.93,69.85 MODUL1.13
N$87  (via drill 0.61)
  Top 0.305: v97.79,60.33 97.79,73.03 96.52,74.3 96.52,78.74 96.2,79.06 96.2,80.64 94.61,80.64 93.66,79.69 93.66,78.74 DZ6.20 | v83.82,57.47 74.61,66.67 MODUL1.14
  Bottom 0.305: v97.79,60.33 94.93,57.47 v83.82,57.47
N$88
  Top 0.305: DZ5.1 RN9.6
N$89
  Top 0.305: RN7.4 DZ4.3
N$90
  Top 0.305: RN7.3 DZ4.4
N$91
  Top 0.305: RN7.2 DZ4.5
N$92
  Top 0.305: RN8.5 DZ4.7
N$93
  Top 0.305: RN8.4 DZ4.8
N$94
  Top 0.305: RN8.3 DZ4.9
N$95
  Top 0.305: RN8.2 DZ4.10
N$104
  Top 0.305: RN7.6 DZ4.1
N$105
  Top 0.305: RN7.5 DZ4.2
N$106
  Top 0.305: RN8.6 112.08,5.08 113.03,6.03 113.03,11.75 112.08,12.7 DZ4.6
N$109
  Top 0.305: DZ5.2 RN9.5
N$110
  Top 0.305: DZ5.6 RN10.6
N$113
  Top 0.305: DZ6.3 RN11.4
N$114
  Top 0.305: DZ6.4 RN11.3
N$115
  Top 0.305: DZ6.5 RN11.2
N$116
  Top 0.305: DZ6.7 RN12.5
N$117
  Top 0.305: DZ6.8 RN12.4
N$118
  Top 0.305: DZ6.9 RN12.3
N$119
  Top 0.305: DZ6.10 RN12.2
N$120  (via drill 0.61)
  Top 0.305: MODUL1.17 v74.93,75.56
  Bottom 0.305: v74.93,75.56 84.77,75.56 85.72,76.52 DZ6.17
N$121  (via drill 0.61)
  Top 0.305: v94.93,79.38 95.89,78.42 95.89,73.66 94.93,72.71 94.93,60.96 95.57,60.33 v95.57,59.69 | v77.47,58.74 69.53,66.67 MODUL1.18
  Bottom 0.305: v94.93,79.38 85.41,79.38 84.45,78.42 DZ6.16 | v95.57,59.69 94.61,58.74 v77.47,58.74
N$122  (via drill 0.61)
  Top 0.305: v70.48,81.92 68.58,80.01 68.58,72.39 66.67,70.48 MODUL1.19
  Bottom 0.305: v70.48,81.92 77.15,81.92 80.64,78.42 DZ6.15
N$123  (via drill 0.61)
  Top 0.305: v76.2,97.79 82.55,91.44 82.55,83.82 80.64,81.92 80.64,80.33 79.06,78.74 DZ6.14 | v12.38,95.25 10.48,93.34 10.48,84.45 9.21,83.19 ISP1.7 8.57,81.92 7.62,80.96 7.62,74.3 3.17,69.85 3.17,21.59 6.03,21.59 6.99,22.54 ATMEL.3 | v64.45,60.96 64.45,64.77 66.36,66.67 MODUL1.20
  Bottom 0.305: v76.2,97.79 75.56,98.42 15.56,98.42 v12.38,95.25 | v64.45,60.96 59.37,55.88 17.46,55.88 10.16,63.18 10.16,81.92 9.21,81.92 ISP1.7
N$124  (via drill 0.61)
  Top 0.305: 66.04,83.19 70.8,83.19 75.56,78.42 DZ6.13 | 66.04,83.19 66.04,72.39 64.14,70.48 MODUL1.21 | ISP1.1 8.57,74.3 3.81,69.53 3.81,24.45 4.76,23.5 ATMEL.4 | 66.04,83.19 63.5,83.19 v63.5,86.68
  Bottom 0.305: v63.5,86.68 56.83,93.34 40.64,93.34 40.01,93.98 11.43,93.98 7.62,90.17 7.62,75.56 8.57,75.56 ISP1.1
N$125  (via drill 0.61)
  Top 0.305: 12.06,60.01 v12.06,81.92 | 12.06,60.01 12.06,25.08 7.94,20.95 ATMEL.1 | v63.18,61.28 63.18,66.04 63.82,66.67 MODUL1.22 | 12.06,60.01 v19.05,60.01
  Bottom 0.305: 12.06,82.55 11.75,82.55 9.53,84.77 ISP1.9 | 12.06,82.55 30.16,82.55 32.07,80.64 70.8,80.64 73.03,78.42 DZ6.12 | v12.06,81.92 12.06,82.55 | v63.18,61.28 61.91,60.01 v19.05,60.01
N$126
  Bottom 0.305: DZ6.11 70.48,78.42 69.53,79.38 56.52,79.38 55.88,78.74 55.88,71.12 60.01,71.12 60.96,70.17 MODUL1.23
N$128
  Top 0.305: DZ6.1 RN11.6
N$129
  Top 0.305: DZ6.2 RN11.5
N$130
  Top 0.305: DZ6.6 RN12.6
N$131  (via drill 0.61)
  Top 0.305: v98.42,81.92 101.6,78.74 101.6,60.64 v94.61,53.66 | v84.45,53.66 72.07,66.04 72.07,66.67 MODUL1.16 | v88.9,81.92 DZ6.18
  Bottom 0.305: v98.42,81.92 v88.9,81.92 | v84.45,53.66 v94.61,53.66
N$132  (via drill 0.61)
  Top 0.305: v90.17,83.19 90.17,79.69 91.12,78.74 DZ6.19 | v80.33,83.19 77.47,80.33 77.47,76.2 71.75,70.48 MODUL1.15
  Bottom 0.305: v80.33,83.19 v90.17,83.19
N$133
  Top 0.305: DZ7.3 RN13.4
N$134
  Top 0.305: DZ7.4 RN13.3
N$135
  Top 0.305: DZ7.5 57.47,86.36 58.42,87.31 58.42,94.3 57.47,95.25 RN13.2
N$136
  Top 0.305: DZ7.7 52.39,86.36 54.29,88.27 54.29,88.9 RN14.5
N$137
  Top 0.305: DZ7.8 49.85,86.36 51.75,88.27 51.75,88.9 RN14.4
N$138
  Top 0.305: DZ7.9 47.31,86.36 49.21,88.27 49.21,88.9 RN14.3
N$139
  Top 0.305: DZ7.10 44.77,86.36 46.67,88.27 46.67,88.9 RN14.2
N$140
  Top 0.305: DZ7.17 59.37,76.2 56.52,73.34 56.52,70.48 MODUL1.27
N$142  (via drill 0.61)
  Top 0.305: v96.52,72.71 96.2,72.39 v96.2,61.91
  Bottom 0.305: v96.52,72.71 95.25,72.71 93.66,74.3 92.71,74.3 92.08,73.66 69.85,73.66 68.9,74.61 59.69,74.61 57.78,76.52 DZ7.16 | v96.2,61.91 95.57,61.28 93.98,61.28 93.34,60.64 67.94,60.64 66.04,62.55 56.52,62.55 52.07,66.99 MODUL1.32
N$143  (via drill 0.61)
  Top 0.305: v50.48,72.39 48.9,70.8 48.9,70.48 MODUL1.33
  Bottom 0.305: v50.48,72.39 54.29,76.2 DZ7.15
N$144  (via drill 0.61)
  Top 0.305: v22.86,80.64 21.59,79.38 v21.59,66.67
  Bottom 0.305: v22.86,80.64 24.45,80.64 25.08,80.01 49.85,80.01 51.44,78.42 DZ7.14 | v21.59,66.67 25.72,62.55 43.81,62.55 48.26,66.99 MODUL1.34
N$145
  Top 0.305: DZ7.13 49.21,76.2 46.35,73.34 46.35,70.48 MODUL1.35
N$146  (via drill 0.61)
  Top 0.305: v26.04,73.34 25.08,72.39 25.08,66.99 v28.26,63.82
  Bottom 0.305: v26.04,73.34 26.67,73.34 26.99,73.03 42.86,73.03 46.35,76.52 DZ7.12 | v28.26,63.82 28.89,64.45 43.18,64.45 45.72,66.99 MODUL1.36
N$147
  Top 0.305: DZ7.11 44.13,76.2 43.81,75.88 43.81,70.48 MODUL1.37
N$148
  Top 0.305: DZ7.1 RN13.6
N$149
  Top 0.305: DZ7.2 RN13.5
N$150
  Top 0.305: DZ7.6 54.93,86.36 56.83,88.27 56.83,88.9 RN14.6
N$153
  Top 0.305: DZ8.3 35.88,86.36 36.83,87.31 36.83,94.3 35.88,95.25 RN15.4
N$154
  Top 0.305: DZ8.4 33.34,86.36 34.29,87.31 34.29,94.3 33.34,95.25 RN15.3
N$155
  Top 0.305: DZ8.5 30.16,86.36 29.21,87.31 29.21,94.3 30.16,95.25 RN15.2
N$156
  Bottom 0.305: DZ8.7 26.04,86.04 28.26,88.27 33.97,88.27 34.92,89.22 RN16.5
N$157
  Bottom 0.305: DZ8.8 23.5,84.14 24.45,83.19 38.73,83.19 39.37,83.82 39.37,92.08 34.61,92.08 33.66,91.12 RN16.4
N$158
  Top 0.305: DZ8.9 20.95,84.14 21.91,83.19 31.75,83.19 31.75,87.95 30.8,88.9 RN16.3
N$159
  Bottom 0.305: DZ8.10 18.41,86.04 20.64,88.27 26.35,88.27 27.3,89.22 RN16.2
N$160  (via drill 0.61)
  Top 0.305: v22.86,61.28 v22.86,72.07 | v37.15,61.28 40.96,65.09 40.96,66.67 MODUL1.40
  Bottom 0.305: v22.86,72.07 26.35,75.56 33.97,75.56 34.92,76.52 DZ8.18 | v22.86,61.28 v37.15,61.28
N$161
  Top 0.305: DZ8.17 33.34,76.2 38.42,71.12 38.42,70.48 MODUL1.41
N$163  (via drill 0.61)
  Top 0.305: v28.89,74.3 28.89,75.56 28.26,76.2 DZ8.15 | v31.43,74.3 35.56,70.17 MODUL1.43
  Bottom 0.305: v28.89,74.3 v31.43,74.3
N$164  (via drill 0.61)
  Top 0.305: v21.27,80.64 21.27,81.92 23.18,81.92 25.4,79.69 DZ8.14 | v34.61,58.74 35.88,60.01 35.88,66.67 MODUL1.44
  Bottom 0.305: v21.27,80.64 21.27,79.06 21.59,78.74 21.59,73.66 18.73,73.66 17.78,72.71 17.78,58.74 v34.61,58.74
N$165
  Bottom 0.305: DZ8.13 22.54,76.2 22.54,73.34 21.59,72.39 21.59,70.8 27.62,70.8 27.94,71.12 32.07,71.12 33.02,70.17 MODUL1.45
N$166  (via drill 0.61)
  Top 0.305: v32.38,57.15 33.34,58.1 33.34,66.67 MODUL1.46
  Bottom 0.305: v32.38,57.15 17.14,57.15 17.14,73.34 20,76.2 DZ8.12
N$167
  Top 0.305: DZ8.11 17.78,80.33 20,82.55 31.75,82.55 31.75,76.2 30.16,74.61 30.16,71.12 30.8,70.48 MODUL1.47
N$168
  Top 0.305: DZ8.1 RN15.6
N$169
  Top 0.305: DZ8.2 38.42,86.36 39.37,87.31 39.37,94.3 38.42,95.25 RN15.5
N$170
  Bottom 0.305: DZ8.6 28.57,86.04 30.16,87.63 35.88,87.63 37.47,89.22 RN16.6
N$171
  Top 0.305: DZ8.19 38.42,76.2 40.96,73.66 40.96,70.48 MODUL1.39
N$172  (via drill 0.61)
  Top 0.305: v24.13,65.72 v24.13,79.38
  Bottom 0.305: v24.13,79.38 39.05,79.38 40.01,78.42 DZ8.20 | v24.13,65.72 24.77,65.09 41.27,65.09 43.18,66.99 MODUL1.38
PA0  (via drill 0.61)
  Top 0.305: v93.34,17.14 96.52,20.32 96.52,33.34 v95.89,33.97 | v60.01,37.47 59.37,36.83 59.37,32.07 MODUL1.76 | v80.01,18.41 DZ3.17
  Bottom 0.305: v80.01,18.41 81.28,17.14 v93.34,17.14 | v95.89,33.97 93.66,36.2 90.81,36.2 89.53,37.47 v60.01,37.47
PA1  (via drill 0.61)
  Top 0.305: v64.77,17.78 62.23,20.32 62.23,23.18 59.05,26.35 59.05,28.57 MODUL1.75 | v77.47,18.41 DZ3.18
  Bottom 0.305: v77.47,18.41 76.83,17.78 v64.77,17.78
PA2  (via drill 0.61)
  Top 0.305: v91.12,19.68 91.44,20 91.44,26.35 92.71,27.62 v92.71,33.97
  Bottom 0.305: v91.12,19.68 76.52,19.68 75.56,20.64 DZ3.19 | v92.71,33.97 92.39,33.66 88.9,33.66 88.27,34.29 59.69,34.29 57.15,31.75 MODUL1.74
PA3  (via drill 0.61)
  Top 0.305: v69.22,25.72 72.07,22.86 DZ3.20
  Bottom 0.305: v69.22,25.72 67.94,26.99 61.59,26.99 60.64,27.94 60.01,27.94 59.69,27.62 58.42,27.62 57.15,28.89 MODUL1.73
PA4  (via drill 0.61)
  Top 0.305: v87,24.45 90.81,28.26 90.81,33.97 89.22,35.56 v89.22,36.2
  Bottom 0.305: v87,24.45 73.66,24.45 73.03,23.81 70.48,23.81 69.22,22.54 DZ2.11 | v89.22,36.2 54.93,36.2 53.98,35.24 53.98,32.07 MODUL1.72
PA5  (via drill 0.61)
  Top 0.305: v60.33,26.67 62.55,24.45 62.55,23.81 64.14,23.81 65.41,22.54 DZ2.12
  Bottom 0.305: v60.33,26.67 60.01,26.99 56.52,26.99 54.61,28.89 MODUL1.71
PA6  (via drill 0.61)
  Top 0.305: v89.85,25.72 91.44,27.3 v91.44,34.92 | v55.24,34.92 52.07,31.75 MODUL1.70
  Bottom 0.305: v89.85,25.72 73.98,25.72 72.71,24.45 66.04,24.45 64.14,22.54 DZ2.13 | v55.24,34.92 v91.44,34.92
PA7
  Top 0.305: DZ2.14 60.33,22.54 55.24,27.62 51.75,27.62 51.75,28.57 MODUL1.69
PB5  (via drill 0.61)
  Top 0.305: v94.61,74.93 94.3,74.61 v94.3,60.01 | v66.36,59.69 61.91,59.69 61.91,66.67 MODUL1.24
  Bottom 0.305: v94.61,74.93 92.39,74.93 91.76,74.3 70.17,74.3 67.94,76.52 DZ7.20 | v94.3,60.01 66.67,60.01 v66.36,59.69
PB6
  Top 0.305: DZ7.19 64.45,76.2 63.5,75.25 63.5,73.03 61.59,71.12 59.05,71.12 59.05,70.48 MODUL1.25
PB7  (via drill 0.61)
  Top 0.305: v93.03,61.91 v93.03,73.03 | v59.69,63.82 59.37,64.14 59.37,66.67 MODUL1.26 | v62.23,73.34 DZ7.18
  Bottom 0.305: v62.23,73.34 62.55,73.03 v93.03,73.03 | v93.03,61.91 92.39,62.55 69.53,62.55 68.26,63.82 v59.69,63.82
PC0  (via drill 0.61)
  Top 0.305: v24.45,28.26 24.45,22.86 DZ1.18
  Bottom 0.305: v24.45,28.26 25.08,27.62 29.21,27.62 30.48,28.89 MODUL1.53
PC1  (via drill 0.61)
  Top 0.305: v21.59,24.13 22.23,24.77 22.23,35.88 21.59,36.51 21.59,37.15 23.81,39.37 30.48,39.37 30.48,32.07 MODUL1.54
  Bottom 0.305: v21.59,24.13 24.45,24.13 26.04,22.54 DZ1.17
PC2  (via drill 0.61)
  Top 0.305: v31.75,24.13 33.34,25.72 33.34,28.57 MODUL1.55
  Bottom 0.305: v31.75,24.13 31.43,24.13 29.84,22.54 DZ1.16
PC3  (via drill 0.61)
  Top 0.305: v26.99,32.38 26.99,27.3 31.43,22.86 DZ1.15
  Bottom 0.305: v26.99,32.38 27.62,33.02 32.07,33.02 33.02,32.07 MODUL1.56
PC4
  Top 0.305: DZ1.14 34.61,22.86 35.88,24.13 35.88,28.57 MODUL1.57
PC5  (via drill 0.61)
  Top 0.305: v25.72,35.24 25.72,27.62 27.94,25.4 27.94,19.68 35.24,19.68 36.2,20.64 DZ1.13 | v32.38,35.24 35.56,32.07 MODUL1.58
  Bottom 0.305: v25.72,35.24 v32.38,35.24
PC6
  Top 0.305: DZ1.12 39.05,22.86 39.05,28.57 MODUL1.59
PC7  (via drill 0.61)
  Top 0.305: v22.86,36.83 22.86,19.05 39.69,19.05 41.27,20.64 DZ1.11 | v33.34,36.83 38.1,32.07 MODUL1.60
  Bottom 0.305: v22.86,36.83 v33.34,36.83
PE0  (via drill 0.61)
  Top 0.305: v109.22,68.26 117.47,76.52 DZ5.19
  Bottom 0.305: v109.22,68.26 108.27,67.31 90.17,67.31 MODUL1.2
PE1  (via drill 0.61)
  Top 0.305: v97.47,80.64 96.84,81.28 92.71,81.28 92.71,76.2 87,70.48 MODUL1.3
  Bottom 0.305: v97.47,80.64 112.71,80.64 114.94,78.42 DZ5.18
PE2  (via drill 0.61)
  Top 0.305: v105.41,61.91 105.41,68.9 112.71,76.2 DZ5.17 | v90.49,54.93 87.31,58.1 87.31,66.67 MODUL1.4
  Bottom 0.305: v105.41,61.91 98.42,54.93 v90.49,54.93
PE3
  Top 0.305: DZ5.16 109.86,78.42 105.09,83.19 92.71,83.19 92.71,97.79 92.08,98.42 85.09,98.42 85.09,69.85 MODUL1.5
PE4  (via drill 0.61)
  Top 0.305: v104.14,66.04 104.14,72.71 107.63,76.2 DZ5.15
  Bottom 0.305: v104.14,66.04 103.82,66.36 90.49,66.36 89.85,65.72 86.36,65.72 85.09,66.99 MODUL1.6
PE6  (via drill 0.61)
  Top 0.305: v102.87,61.91 102.87,73.98 105.09,76.2 DZ5.14 | v87,56.2 82.23,60.96 82.23,66.67 MODUL1.8
  Bottom 0.305: v102.87,61.91 97.16,56.2 v87,56.2
PE7  (via drill 0.61)
  Top 0.305: v81.92,80.64 80.01,78.74 80.01,69.85 MODUL1.9
  Bottom 0.305: v81.92,80.64 95.25,80.64 96.52,79.38 101.28,79.38 102.23,78.42 DZ5.13
PF1  (via drill 0.61)
  Top 0.305: v111.12,32.7 121.28,22.54 DZ4.11 | v87.95,33.02 82.23,33.02 82.23,32.07 MODUL1.94
  Bottom 0.305: v111.12,32.7 90.49,32.7 90.17,33.02 v87.95,33.02
PF2
  Top 0.305: DZ4.12 118.75,20.64 117.79,19.68 115.57,19.68 115.57,22.86 114.94,23.5 107.95,23.5 107.95,20.32 103.5,15.88 91.44,15.88 91.44,2.54 90.81,1.91 83.82,1.91 83.82,26.99 82.23,28.57 MODUL1.93
PF3  (via drill 0.61)
  Top 0.305: v102.87,36.51 116.52,22.86 DZ4.13 | v91.12,37.47 79.69,37.47 79.69,32.07 MODUL1.92
  Bottom 0.305: v102.87,36.51 101.92,37.47 v91.12,37.47
PF4
  Top 0.305: DZ4.14 113.98,20.32 110.49,16.83 110.49,7.62 104.14,1.27 81.28,1.27 81.28,26.04 79.69,27.62 79.69,28.57 MODUL1.91
PF5  (via drill 0.61)
  Top 0.305: v95.25,25.08 94.61,25.72 94.61,37.47 91.12,40.96 76.83,40.96 76.83,32.07 MODUL1.90
  Bottom 0.305: v95.25,25.08 108.58,25.08 111.12,22.54 DZ4.15
PF6  (via drill 0.61)
  Top 0.305: v80.01,5.71 78.74,6.99 78.74,26.99 77.15,28.57 MODUL1.89
  Bottom 0.305: v80.01,5.71 105.41,5.71 105.41,15.24 106.05,15.88 108.9,15.88 108.9,20.32 DZ4.16
PF7  (via drill 0.61)
  Top 0.305: v101.6,43.81 101.6,27.62 106.36,22.86 DZ4.17 | v77.79,44.13 74.61,40.96 74.61,32.07 MODUL1.88
  Bottom 0.305: v101.6,43.81 100.65,44.77 78.42,44.77 v77.79,44.13
PG2  (via drill 0.61)
  Top 0.305: v53.66,16.51 57.78,20.64 DZ2.15
  Bottom 0.305: v53.66,16.51 13.34,16.51 8.26,21.59 4.45,21.59 3.17,22.86 3.17,36.83 20,36.83 22.54,39.37 40.96,39.37 48.26,32.07 MODUL1.68
PH0  (via drill 0.61)
  Top 0.305: v99.06,65.09 99.06,75.25 100.01,76.2 DZ5.12 | v80.64,65.72 77.15,65.72 77.15,66.67 MODUL1.12
  Bottom 0.305: v99.06,65.09 81.28,65.09 v80.64,65.72
PJ5  (via drill 0.61)
  Top 0.305: v50.8,17.78 50.8,18.1 53.02,20.32 DZ2.17
  Bottom 0.305: MODUL1.66 45.72,32.07 39.69,38.1 R2.2 22.23,38.1 20.32,36.2 3.81,36.2 3.81,24.77 4.45,24.13 8.26,24.13 13.97,18.41 50.16,18.41 v50.8,17.78
PJ6
  Top 0.305: DZ2.16 55.24,22.54 49.21,28.57 MODUL1.67
PJ7  (via drill 0.61)
  Top 0.305: v81.92,26.99 81.92,23.18 82.23,22.86 DZ3.16
  Bottom 0.305: v81.92,26.99 81.28,27.62 63.5,27.62 62.23,28.89 MODUL1.77
PK0  (via drill 0.61)
  Top 0.305: v76.52,6.99 76.2,7.3 76.2,26.99 74.61,28.57 MODUL1.87
  Bottom 0.305: v76.52,6.99 100.33,6.99 100.33,15.24 100.97,15.88 103.82,15.88 103.82,20.32 DZ4.18
PK1  (via drill 0.61)
  Top 0.305: v100.33,43.5 100.33,23.81 101.28,22.86 DZ4.19 | v72.71,42.86 72.07,42.23 72.07,32.07 MODUL1.86
  Bottom 0.305: v100.33,43.5 99.69,42.86 v72.71,42.86
PK2  (via drill 0.61)
  Top 0.305: v73.66,10.79 73.66,26.99 72.07,28.57 MODUL1.85
  Bottom 0.305: v73.66,10.79 96.52,10.79 96.52,13.97 98.42,15.88 98.74,15.88 98.74,20.32 DZ4.20
PK3  (via drill 0.61)
  Top 0.305: v78.11,39.69 91.44,39.69 93.98,37.15 93.98,23.81 94.93,22.86 DZ3.11 | v70.48,39.37 69.53,38.42 69.53,32.07 MODUL1.84
  Bottom 0.305: v78.11,39.69 77.79,39.37 v70.48,39.37
PK4  (via drill 0.61)
  Top 0.305: v71.44,15.88 69.85,17.46 69.85,23.5 67.94,25.4 67.94,27.62 68.9,28.57 MODUL1.83
  Bottom 0.305: v71.44,15.88 97.47,15.88 97.47,18.73 96.52,19.68 94.3,19.68 93.34,20.64 DZ3.12
PK5  (via drill 0.61)
  Top 0.305: v97.79,26.35 97.16,26.99 97.16,41.27 92.71,45.72 66.99,45.72 66.99,32.07 MODUL1.82
  Bottom 0.305: v97.79,26.35 94.61,26.35 90.81,22.54 DZ3.13
PK6  (via drill 0.61)
  Top 0.305: v88.9,12.38 88.9,19.37 87.95,20.32 DZ3.14 | v67.31,12.06 67.31,28.89 MODUL1.81
  Bottom 0.305: v88.9,12.38 88.58,12.06 v67.31,12.06

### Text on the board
tPlace: 1 | - | + | V.1.2 | www.robotikhardware.de | + | - | 6 | Testboard für RN-Mega2560 | ISP | 1 | Power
